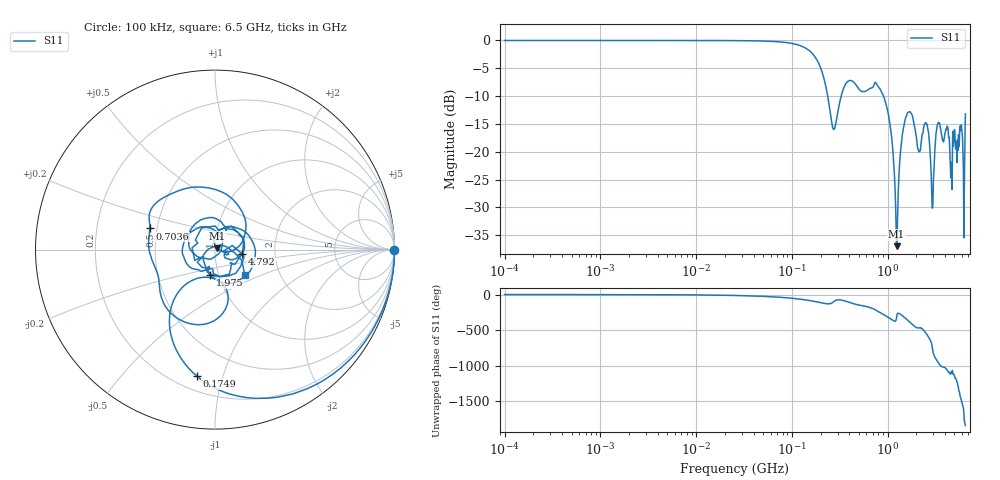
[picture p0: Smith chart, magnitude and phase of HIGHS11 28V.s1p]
!Keysight Technologies,E5080B,MY59100498,A.17.05.10
!Date: Wednesday, August 30, 2023 19:24:56
!Correction: S11(C  1-Port  )
!S1P File: Measurement: S11:Log Frequency Sweep
# Hz S  dB  R 50
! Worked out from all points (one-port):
!   1601 points, 100 kHz to 6.5 GHz, reference 50 ohm
!   lowest |S11| = -37.0 dB at 1.242 GHz (marker M1), VSWR 1.03, Z = 51.2 + j0.833 ohm
!   |S11| at or under -10 dB: 236.9 MHz to 327.6 MHz (90.74 MHz wide, 32.1 % of centre); 907.5 MHz to end of sweep
!   S11 on the Smith chart (normalised r, x): 100 kHz: open; 174.9 MHz: 0.29, -0.82; 703.6 MHz: 0.46, +0.13; 1.975 GHz: 0.91, -0.27; 4.792 GHz: 1.35, -0.06; 6.5 GHz: 1.33, -0.40
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100000  -0.00 -0.1
399589.6  -0.00 -0.2
1596718  -0.01 -0.8
6380321  -0.00 -3.1
2.54951e7  -0.03 -12.7
5.894314e7  -0.15 -29.9
1.018758e8  -0.55 -53.3
1.74864e8  -2.96 -98.3
2.167457e8  -6.85 -123.9
2.724062e8  -15.97 -103.2
3.28424e8  -9.93 -78.0
4.070849e8  -7.18 -114.0
7.035948e8  -8.37 162.0
8.366126e8  -8.76 107.0
1.008654e9  -12.84 41.2
1.111361e9  -17.89 5.7
1.241608e9  -36.96 35.0
1.416243e9  -17.36 66.1
1.626669e9  -12.95 -2.1
1.974809e9  -16.76 -100.7
2.145962e9  -19.89 -108.5
2.551666e9  -15.03 165.2
2.930793e9  -30.13 -24.4
3.389649e9  -14.83 121.7
4.172505e9  -15.40 22.1
4.792457e9  -16.33 -8.8
5.317155e9  -21.92 -150.2
6.5e9  -13.18 -40.7
